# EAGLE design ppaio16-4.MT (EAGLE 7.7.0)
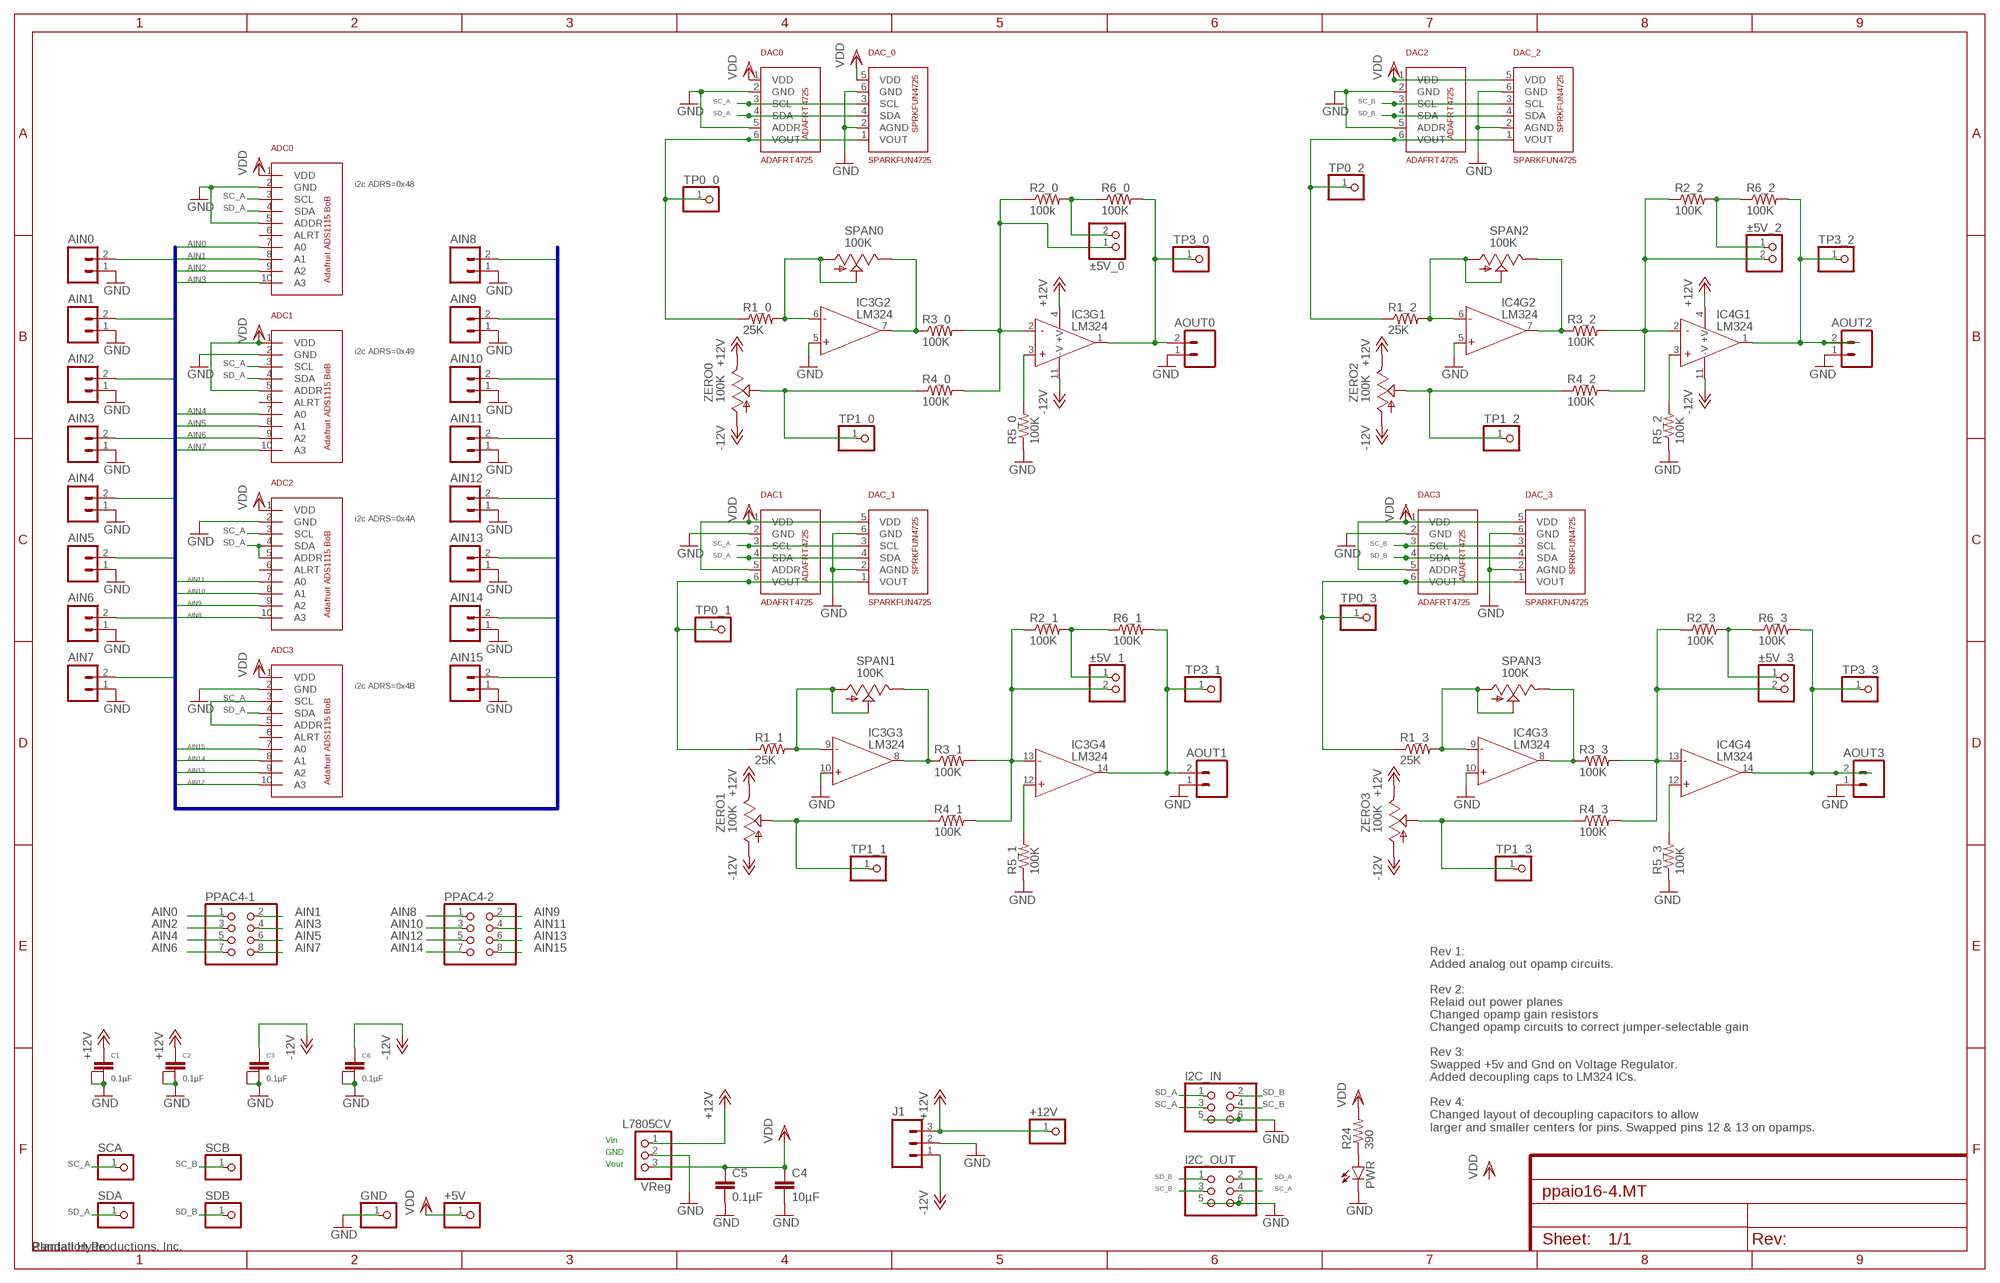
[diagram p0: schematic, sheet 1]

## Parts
+5V  PINHD-1X1  [1X01]
+12V  PINHD-1X1  [1X01]
ADC0  ADAFRTADS1115  [SIL10]
ADC1  ADAFRTADS1115  [SIL10]
ADC2  ADAFRTADS1115  [SIL10]
ADC3  ADAFRTADS1115  [SIL10]
AIN0  M025MM  [SCREWTERMINAL-5MM-2]
AIN1  M025MM  [SCREWTERMINAL-5MM-2]
AIN2  M025MM  [SCREWTERMINAL-5MM-2]
AIN3  M025MM  [SCREWTERMINAL-5MM-2]
AIN4  M025MM  [SCREWTERMINAL-5MM-2]
AIN5  M025MM  [SCREWTERMINAL-5MM-2]
AIN6  M025MM  [SCREWTERMINAL-5MM-2]
AIN7  M025MM  [SCREWTERMINAL-5MM-2]
AIN8  M025MM  [SCREWTERMINAL-5MM-2]
AIN9  M025MM  [SCREWTERMINAL-5MM-2]
AIN10  M025MM  [SCREWTERMINAL-5MM-2]
AIN11  M025MM  [SCREWTERMINAL-5MM-2]
AIN12  M025MM  [SCREWTERMINAL-5MM-2]
AIN13  M025MM  [SCREWTERMINAL-5MM-2]
AIN14  M025MM  [SCREWTERMINAL-5MM-2]
AIN15  M025MM  [SCREWTERMINAL-5MM-2]
AOUT0  M025MM  [SCREWTERMINAL-5MM-2]
AOUT1  M025MM  [SCREWTERMINAL-5MM-2]
AOUT2  M025MM  [SCREWTERMINAL-5MM-2]
AOUT3  M025MM  [SCREWTERMINAL-5MM-2]
C1  0.1µF  CAPACITOR  [1+2CAP]
C2  0.1µF  CAPACITOR  [1+2CAP]
C3  0.1µF  CAPACITOR  [1+2CAP]
C4  10µF  C2.5/2  [C2.5-2]
C5  0.1µF  C2.5/2  [C2.5-2]
C6  0.1µF  CAPACITOR  [1+2CAP]
DAC0  ADAFRT4725  [SIL6]
DAC1  ADAFRT4725  [SIL6]
DAC2  ADAFRT4725  [SIL6]
DAC3  ADAFRT4725  [SIL6]
DAC_0  SPARKFUN4725  [SIL6]
DAC_1  SPARKFUN4725  [SIL6]
DAC_2  SPARKFUN4725  [SIL6]
DAC_3  SPARKFUN4725  [SIL6]
FRAME1  FRAME_11X17_CU_MARK  [FR-LTR-ON-PCB]
GND  PINHD-1X1  [1X01]
I2C_IN  PINHD-2X3  [2X03]
I2C_OUT  PINHD-2X3  [2X03]
IC3  LM324  [DIL14]
IC4  LM324  [DIL14]
J1  M03-SCREW-5MM  [SCREWTERMINAL-5MM-3]
L7805CV  VReg  PINHD-1X3  [1X03]
PPAC4-1  PINHD-2X4  [2X04]
PPAC4-2  PINHD-2X4  [2X04]
PWR  LED5MM  [LED5MM]
R1_0  25K  10OHM-1/4W-5%(PTH)  [AXIAL-0.3]
R1_1  25K  10OHM-1/4W-5%(PTH)  [AXIAL-0.3]
R1_2  25K  10OHM-1/4W-5%(PTH)  [AXIAL-0.3]
R1_3  25K  10OHM-1/4W-5%(PTH)  [AXIAL-0.3]
R2_0  100k  10OHM-1/4W-5%(PTH)  [AXIAL-0.3]
R2_1  100K  10OHM-1/4W-5%(PTH)  [AXIAL-0.3]
R2_2  100K  10OHM-1/4W-5%(PTH)  [AXIAL-0.3]
R2_3  100K  10OHM-1/4W-5%(PTH)  [AXIAL-0.3]
R3_0  100K  10OHM-1/4W-5%(PTH)  [AXIAL-0.3]
R3_1  100K  10OHM-1/4W-5%(PTH)  [AXIAL-0.3]
R3_2  100K  10OHM-1/4W-5%(PTH)  [AXIAL-0.3]
R3_3  100K  10OHM-1/4W-5%(PTH)  [AXIAL-0.3]
R4_0  100K  10OHM-1/4W-5%(PTH)  [AXIAL-0.3]
R4_1  100K  10OHM-1/4W-5%(PTH)  [AXIAL-0.3]
R4_2  100K  10OHM-1/4W-5%(PTH)  [AXIAL-0.3]
R4_3  100K  10OHM-1/4W-5%(PTH)  [AXIAL-0.3]
R5_0  100K  10OHM-1/4W-5%(PTH)  [AXIAL-0.3]
R5_1  100K  10OHM-1/4W-5%(PTH)  [AXIAL-0.3]
R5_2  100K  10OHM-1/4W-5%(PTH)  [AXIAL-0.3]
R5_3  100K  10OHM-1/4W-5%(PTH)  [AXIAL-0.3]
R6_0  100K  10OHM-1/4W-5%(PTH)  [AXIAL-0.3]
R6_1  100K  10OHM-1/4W-5%(PTH)  [AXIAL-0.3]
R6_2  100K  10OHM-1/4W-5%(PTH)  [AXIAL-0.3]
R6_3  100K  10OHM-1/4W-5%(PTH)  [AXIAL-0.3]
R24  390  1KOHM-1/4W-1%(PTH)  [AXIAL-0.3]
SCA  PINHD-1X1  [1X01]
SCB  PINHD-1X1  [1X01]
SDA  PINHD-1X1  [1X01]
SDB  PINHD-1X1  [1X01]
SPAN0  100K  TRIM_US-B64Y  [B64Y]
SPAN1  100K  TRIM_US-B64Y  [B64Y]
SPAN2  100K  TRIM_US-B64Y  [B64Y]
SPAN3  100K  TRIM_US-B64Y  [B64Y]
TP0_0  PINHD-1X1  [1X01]
TP0_1  PINHD-1X1  [1X01]
TP0_2  PINHD-1X1  [1X01]
TP0_3  PINHD-1X1  [1X01]
TP1_0  PINHD-1X1  [1X01]
TP1_1  PINHD-1X1  [1X01]
TP1_2  PINHD-1X1  [1X01]
TP1_3  PINHD-1X1  [1X01]
TP3_0  PINHD-1X1  [1X01]
TP3_1  PINHD-1X1  [1X01]
TP3_2  PINHD-1X1  [1X01]
TP3_3  PINHD-1X1  [1X01]
ZERO0  100K  TRIM_US-B64Y  [B64Y]
ZERO1  100K  TRIM_US-B64Y  [B64Y]
ZERO2  100K  TRIM_US-B64Y  [B64Y]
ZERO3  100K  TRIM_US-B64Y  [B64Y]
±5V_0  PINHD-1X2  [1X02]
±5V_1  PINHD-1X2  [1X02]
±5V_2  PINHD-1X2  [1X02]
±5V_3  PINHD-1X2  [1X02]

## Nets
+12V [RelayConn]: +12V.1 C1.1 C2.1 IC3.4(+V) IC4.4(+V) J1.3 L7805CV.1 ZERO0.E ZERO1.E ZERO2.E ZERO3.E
-12V [RelayConn]: C3.1 C6.1 IC3.11(-V) IC4.11(-V) J1.1 ZERO0.A ZERO1.A ZERO2.A ZERO3.A
AIN0: ADC0.7(A0) AIN0.2 PPAC4-1.1
AIN1: ADC0.8(A1) AIN1.2 PPAC4-1.2
AIN2: ADC0.9(A2) AIN2.2 PPAC4-1.3
AIN3: ADC0.10(A3) AIN3.2 PPAC4-1.4
AIN4: ADC1.7(A0) AIN4.2 PPAC4-1.5
AIN5: ADC1.8(A1) AIN5.2 PPAC4-1.6
AIN6: ADC1.9(A2) AIN6.2 PPAC4-1.7
AIN7: ADC1.10(A3) AIN7.2 PPAC4-1.8
AIN8: ADC2.10(A3) AIN8.2 PPAC4-2.1
AIN9: ADC2.9(A2) AIN9.2 PPAC4-2.2
AIN10: ADC2.8(A1) AIN10.2 PPAC4-2.3
AIN11: ADC2.7(A0) AIN11.2 PPAC4-2.4
AIN12: ADC3.10(A3) AIN12.2 PPAC4-2.5
AIN13: ADC3.9(A2) AIN13.2 PPAC4-2.6
AIN14: ADC3.8(A1) AIN14.2 PPAC4-2.7
AIN15: ADC3.7(A0) AIN15.2 PPAC4-2.8
GND [Ground]: ADC0.2(GND) ADC0.5(ADDR) ADC1.2(GND) ADC2.2(GND) ADC3.2(GND) AIN0.1 AIN1.1 AIN2.1 AIN3.1 AIN4.1 AIN5.1 AIN6.1 AIN7.1 AIN8.1 AIN9.1 AIN10.1 AIN11.1 AIN12.1 AIN13.1 AIN14.1 AIN15.1 AOUT0.1 AOUT1.1 AOUT2.1 AOUT3.1 C1.2@1 C1.2@2 C2.2@1 C2.2@2 C3.2@1 C3.2@2 C4.2 C5.2 C6.2@1 C6.2@2 DAC0.2(GND) DAC0.5(ADDR) DAC1.2(GND) DAC2.2(GND) DAC2.5(ADDR) DAC3.2(GND) DAC_0.2(AGND) DAC_0.6(GND) DAC_1.2(AGND) DAC_1.6(GND) DAC_2.2(AGND) DAC_2.6(GND) DAC_3.2(AGND) DAC_3.6(GND) GND.1 I2C_IN.5 I2C_IN.6 I2C_OUT.5 I2C_OUT.6 IC3.5(+IN) IC3.10(+IN) IC4.5(+IN) IC4.10(+IN) J1.2 L7805CV.2 PWR.K(C) R5_0.P$1 R5_1.P$1 R5_2.P$1 R5_3.P$1
N$1: DAC0.6(VOUT) DAC_0.1(VOUT) R1_0.P$1 TP0_0.1
N$2: DAC1.6(VOUT) DAC_1.1(VOUT) R1_1.P$1 TP0_1.1
N$3: DAC2.6(VOUT) DAC_2.1(VOUT) R1_2.P$1 TP0_2.1
N$4: DAC3.6(VOUT) DAC_3.1(VOUT) R1_3.P$1 TP0_3.1
N$5: AOUT0.2 IC3.1(OUT) R6_0.P$2 TP3_0.1
N$6: R2_1.P$2 R6_1.P$1 ±5V_1.1
N$7: R2_3.P$2 R6_3.P$1 ±5V_3.1
N$8: R2_2.P$2 R6_2.P$1 ±5V_2.1
N$9: R2_0.P$2 R6_0.P$1 ±5V_0.2
N$10: IC3.12(+IN) R5_1.P$2
N$11: IC4.12(+IN) R5_3.P$2
N$26: PWR.A R24.P$1
N$38: IC3.6(-IN) R1_0.P$2 SPAN0.A SPAN0.S
N$39: IC3.7(OUT) R3_0.P$1 SPAN0.E
N$40: IC3.2(-IN) R2_0.P$1 R3_0.P$2 R4_0.P$2 ±5V_0.1
N$42: R4_0.P$1 TP1_0.1 ZERO0.S
N$45: IC3.9(-IN) R1_1.P$2 SPAN1.A SPAN1.S
N$46: IC3.8(OUT) R3_1.P$1 SPAN1.E
N$47: IC3.13(-IN) R2_1.P$1 R3_1.P$2 R4_1.P$2 ±5V_1.2
N$48: AOUT1.2 IC3.14(OUT) R6_1.P$2 TP3_1.1
N$49: R4_1.P$1 TP1_1.1 ZERO1.S
N$52: IC3.3(+IN) R5_0.P$2
N$54: IC4.6(-IN) R1_2.P$2 SPAN2.A SPAN2.S
N$55: IC4.7(OUT) R3_2.P$1 SPAN2.E
N$56: IC4.2(-IN) R2_2.P$1 R3_2.P$2 R4_2.P$2 ±5V_2.2
N$57: AOUT2.2 IC4.1(OUT) R6_2.P$2 TP3_2.1
N$58: R4_2.P$1 TP1_2.1 ZERO2.S
N$61: IC4.9(-IN) R1_3.P$2 SPAN3.A SPAN3.S
N$62: IC4.8(OUT) R3_3.P$1 SPAN3.E
N$63: IC4.13(-IN) R2_3.P$1 R3_3.P$2 R4_3.P$2 ±5V_3.2
N$64: AOUT3.2 IC4.14(OUT) R6_3.P$2 TP3_3.1
N$65: R4_3.P$1 TP1_3.1 ZERO3.S
N$68: IC4.3(+IN) R5_2.P$2
SC_A: ADC0.3(SCL) ADC1.3(SCL) ADC2.3(SCL) ADC3.3(SCL) ADC3.5(ADDR) DAC0.3(SCL) DAC1.3(SCL) DAC_0.3(SCL) DAC_1.3(SCL) I2C_IN.3 I2C_OUT.4 SCA.1
SC_B: DAC2.3(SCL) DAC3.3(SCL) DAC_2.3(SCL) DAC_3.3(SCL) I2C_IN.4 I2C_OUT.3 SCB.1
SD_A: ADC0.4(SDA) ADC1.4(SDA) ADC2.4(SDA) ADC2.5(ADDR) ADC3.4(SDA) DAC0.4(SDA) DAC1.4(SDA) DAC_0.4(SDA) DAC_1.4(SDA) I2C_IN.1 I2C_OUT.2 SDA.1
SD_B: DAC2.4(SDA) DAC3.4(SDA) DAC_2.4(SDA) DAC_3.4(SDA) I2C_IN.2 I2C_OUT.1 SDB.1
VDD: +5V.1 ADC0.1(VDD) ADC1.1(VDD) ADC1.5(ADDR) ADC2.1(VDD) ADC3.1(VDD) C4.1 C5.1 DAC0.1(VDD) DAC1.1(VDD) DAC1.5(ADDR) DAC2.1(VDD) DAC3.1(VDD) DAC3.5(ADDR) DAC_0.5(VDD) DAC_1.5(VDD) DAC_2.5(VDD) DAC_3.5(VDD) L7805CV.3 R24.P$2
Unconnected: ADC0.6(ALRT) ADC1.6(ALRT) ADC2.6(ALRT) ADC3.6(ALRT)

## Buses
ABUS:AIN[0..15]

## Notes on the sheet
- i2c ADRS=0x48
- i2c ADRS=0x49
- i2c ADRS=0x4A
- i2c ADRS=0x4B
- Rev 1:
  Added analog out opamp circuits.
  
  Rev 2:
  Relaid out power planes
  Changed opamp gain resistors
  Changed opamp circuits to correct jumper-selectable gain
  
  Rev 3:
  Swapped +5v and Gnd on Voltage Regulator.
  Added decoupling caps to LM324 ICs.
  
  Rev 4:
  Changed layout of decoupling capacitors to allow
  larger and smaller centers for pins. Swapped pins 12 & 13 on opamps.
- Vin
- GND
- Vout

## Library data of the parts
+5V +12V GND SCA SCB SDA SDB TP0_0 TP0_1-TP0_3 TP1_0 TP1_1-TP1_3 TP3_0 TP3_1-TP3_3 = pinhead:PINHD-1X1: PIN HEADER
ADC0 ADC1-ADC3 = PlantProd:ADAFRTADS1115: Adafruit ADS1115 16-bit ADC breakout board
AIN0 AIN1-AIN15 AOUT0 AOUT1-AOUT3 = SparkFun-Connectors:M02: Standard 2-pin 0.1" header. Use with; STOREFRONT_ID: PRT-08432
C1-C3 C6 = PlantProd:CAPACITOR: Capacitor with three terminals to support multiple capacitor sizes.
C4 C5 = capacitor-wima:C: CAPACITOR
DAC0 DAC1-DAC3 = PlantProd:ADAFRT4725: ADAFRT4725 - MCP4725 12-bit DAC BoB
DAC_0 DAC_1-DAC_3 = PlantProd:SPARKFUN4725: ADAFRT4725 - MCP4725 12-bit DAC BoB
FRAME1 = ProperFrame:FRAME_11X17_CU_MARK: Frame sized for 11x17" page with 0.25" margin. Places name, datecode and revision mark in bottom copper layer of PCB.; CNAME: Plantation Productions, Inc.; CREVISION: 2; DESIGNER: Randall Hyde
I2C_IN I2C_OUT = pinhead:PINHD-2X3: PIN HEADER
IC3 IC4 = PlantProd:LM324: LM324 quad op-amp
J1 = SparkFun-Connectors:M03: Header 3 Standard 3-pin 0.1" header. Use with straight break away headers (SKU : PRT-00116), right angle break away headers (PRT-00553), swiss pins (PRT-00743), machine pins (PRT-00117), and female headers (PRT-00115). Molex polarized connector foot print use with SKU : PRT-08232 with associated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; STOREFRONT_ID: PRT-08433
L7805CV = pinhead:PINHD-1X3: PIN HEADER
PPAC4-1 PPAC4-2 = pinhead:PINHD-2X4: PIN HEADER
PWR = SparkFun-LED:LED: LEDs
R1_0 R1_1-R1_3 R2_0 R2_1-R2_3 R3_0 R3_1-R3_3 R4_0 R4_1-R4_3 R5_0 R5_1-R5_3 R6_0 R6_1-R6_3 = SparkFun-Resistors:10OHM-1/4W-5%(PTH): RES-10698; PROD_ID: RES-10698; VALUE: 10
R24 = SparkFun-Resistors:1KOHM-1/4W-1%(PTH): RES-12182; PROD_ID: RES-12182; VALUE: 1K
SPAN0 SPAN1-SPAN3 ZERO0 ZERO1-ZERO3 = pot:TRIM_US-: POTENTIOMETER
±5V_0 ±5V_1-±5V_3 = pinhead:PINHD-1X2: PIN HEADER

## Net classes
1 Ground: width 0.762 mm, drill 1 mm, clearance 0.102 mm
2 RelayConn: width 0.762 mm, drill 0.025 mm, clearance 0.508 mm
3 HiCurSignal: width 0.762 mm, drill 0.025 mm, clearance 0.102 mm

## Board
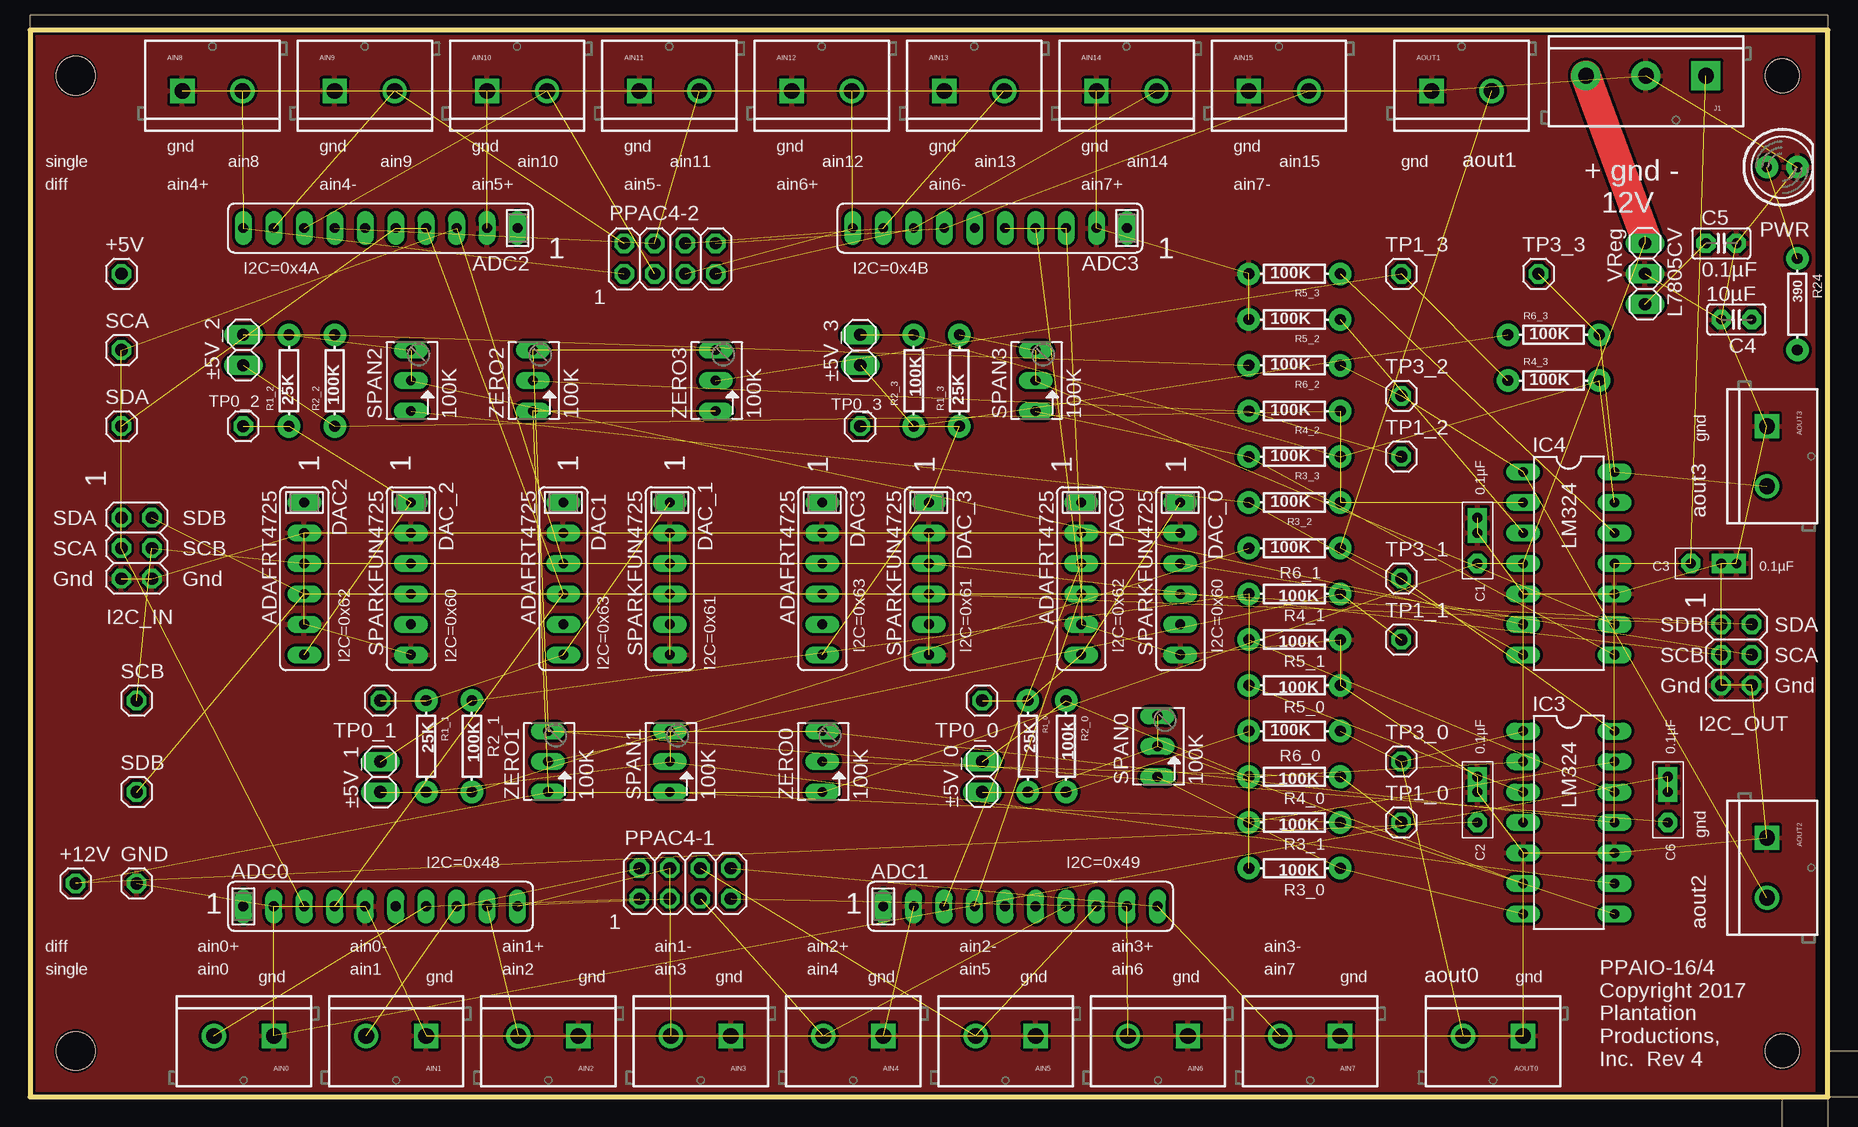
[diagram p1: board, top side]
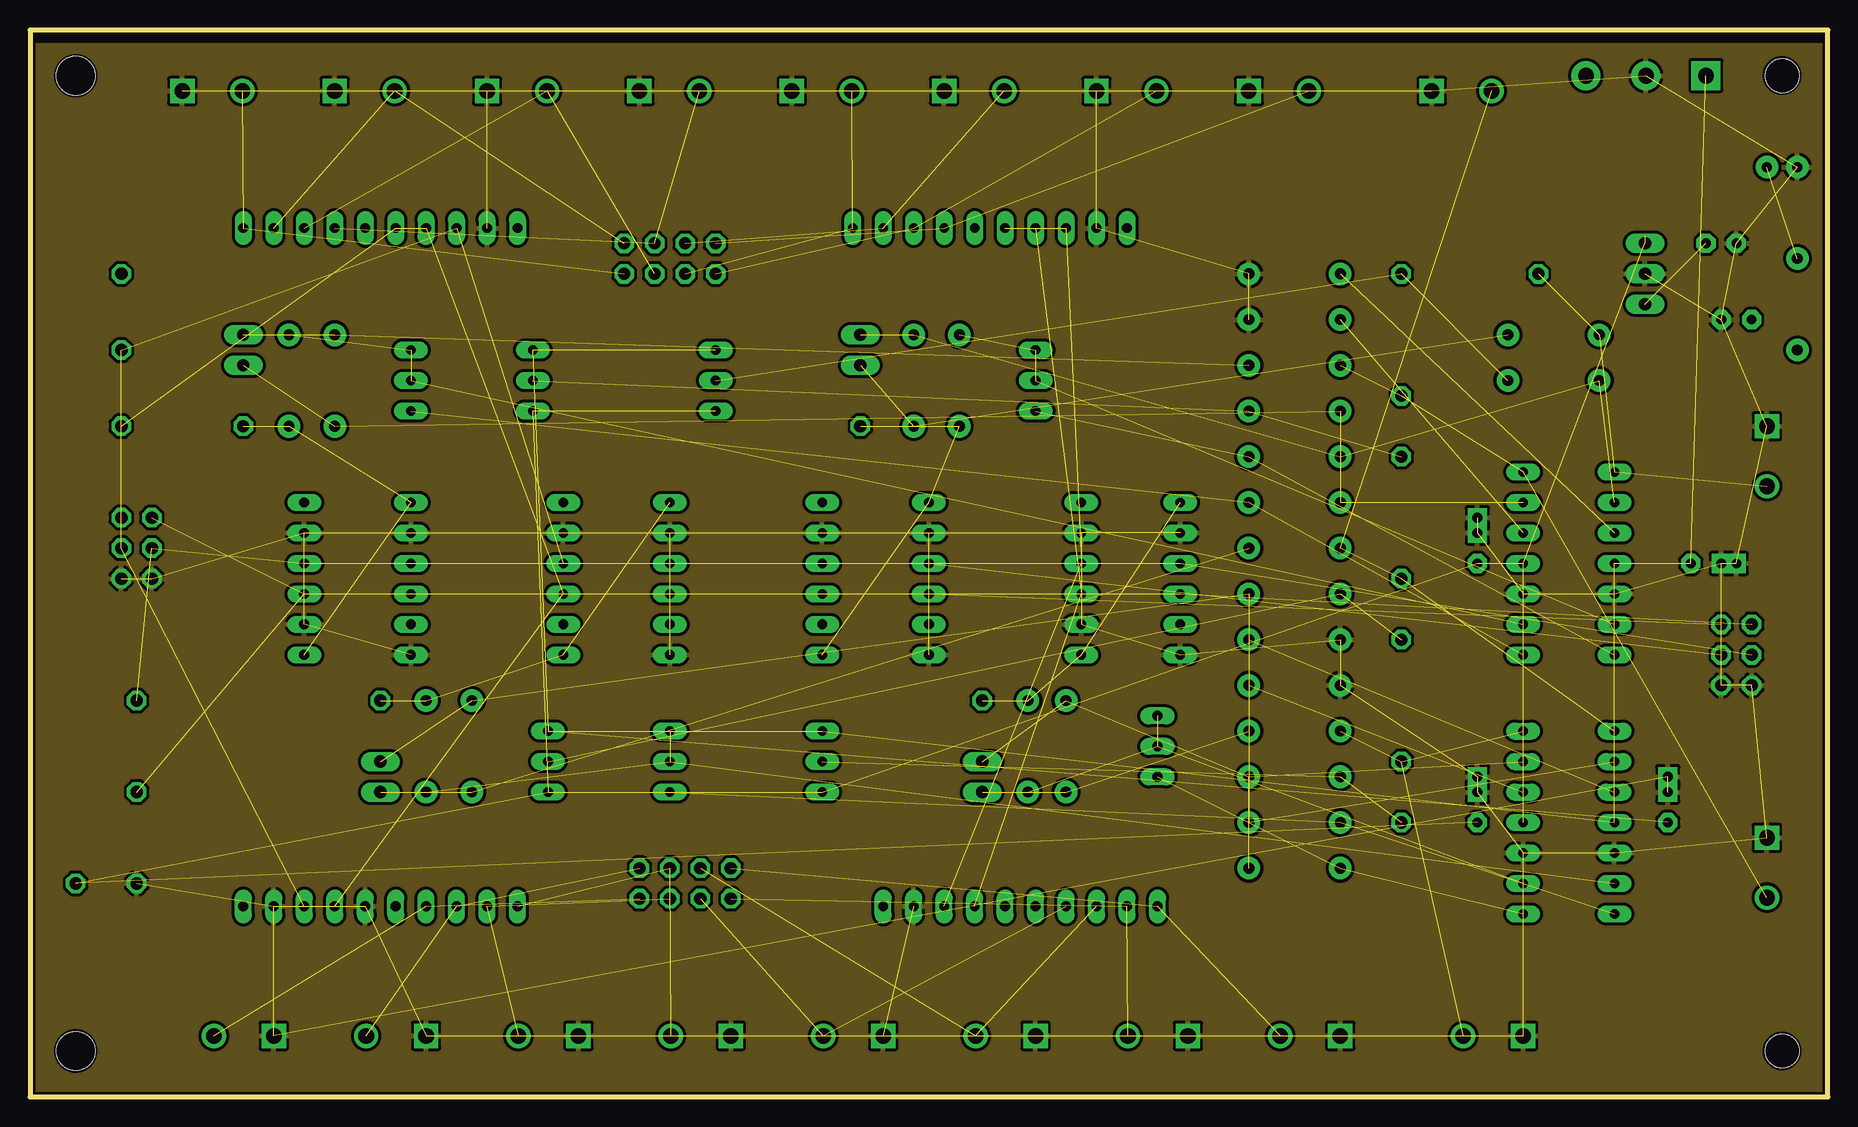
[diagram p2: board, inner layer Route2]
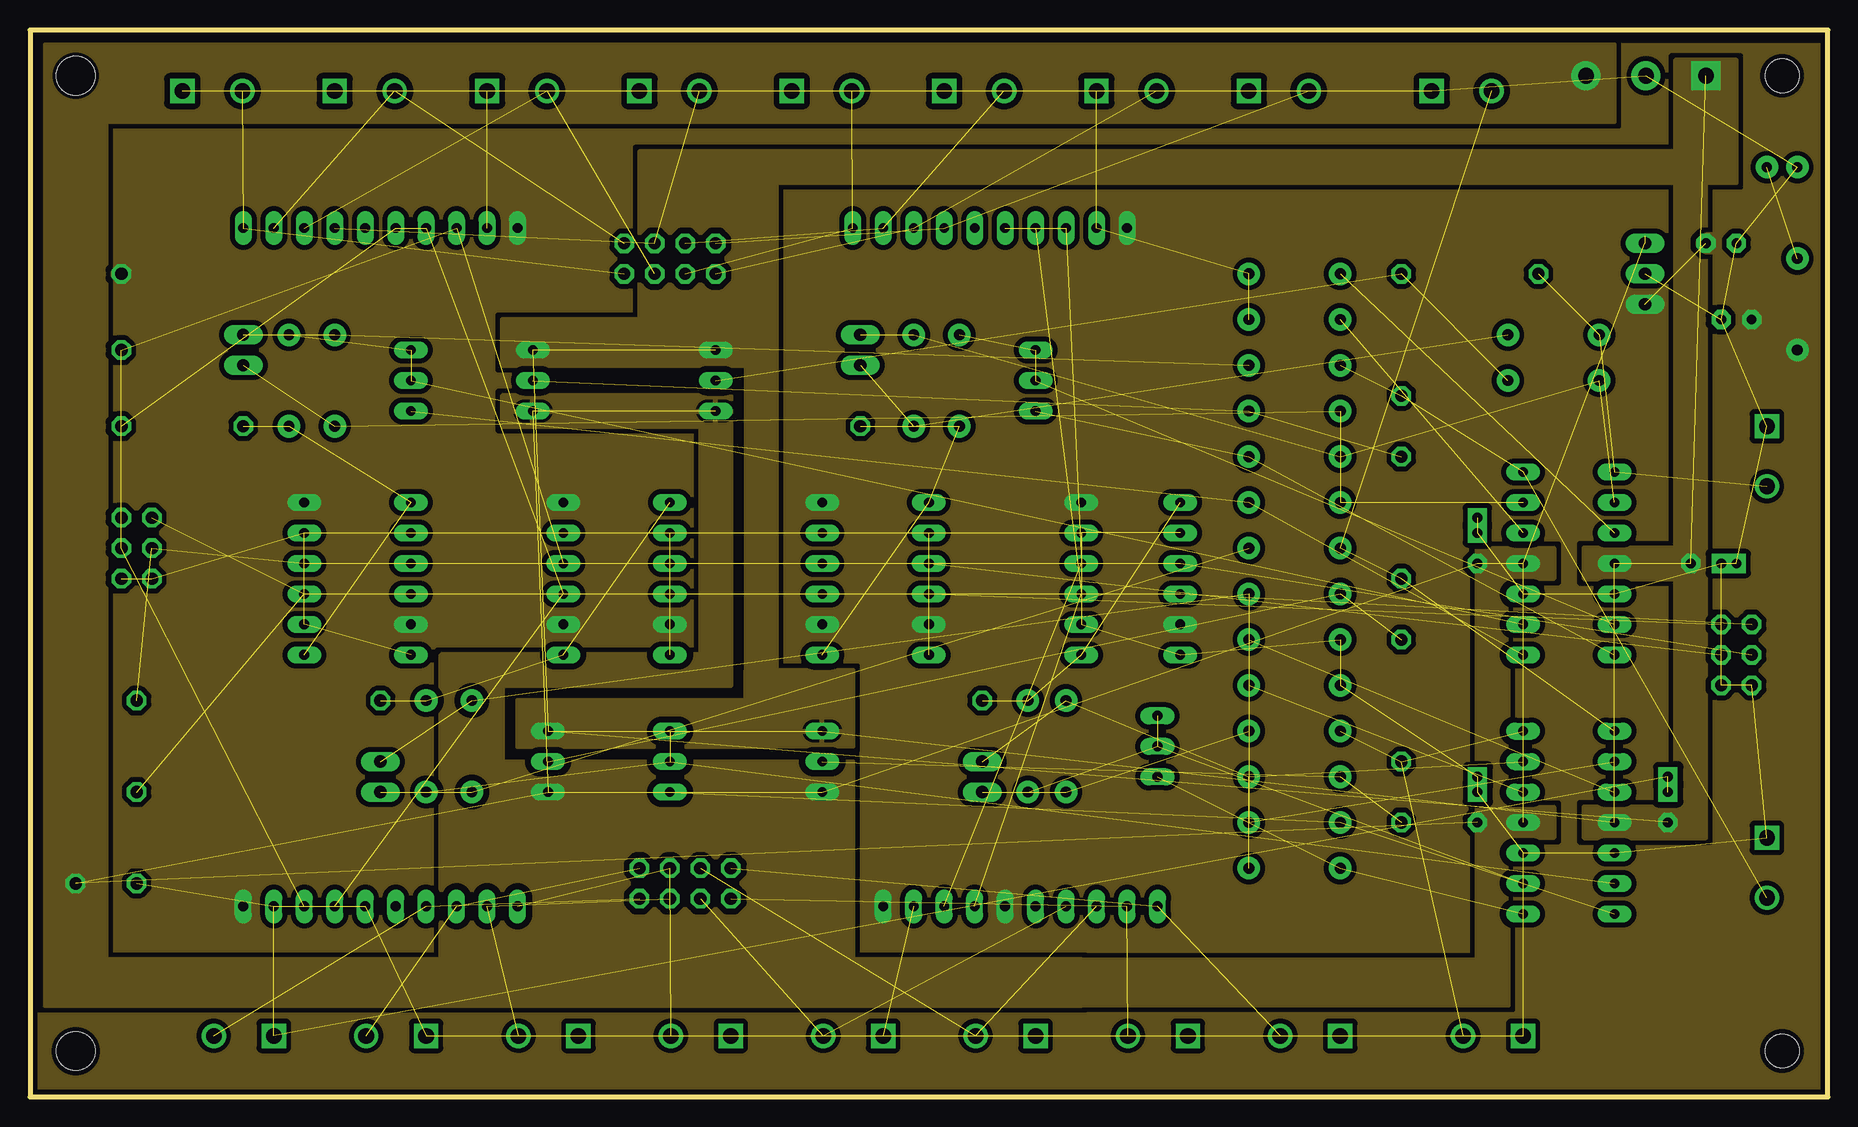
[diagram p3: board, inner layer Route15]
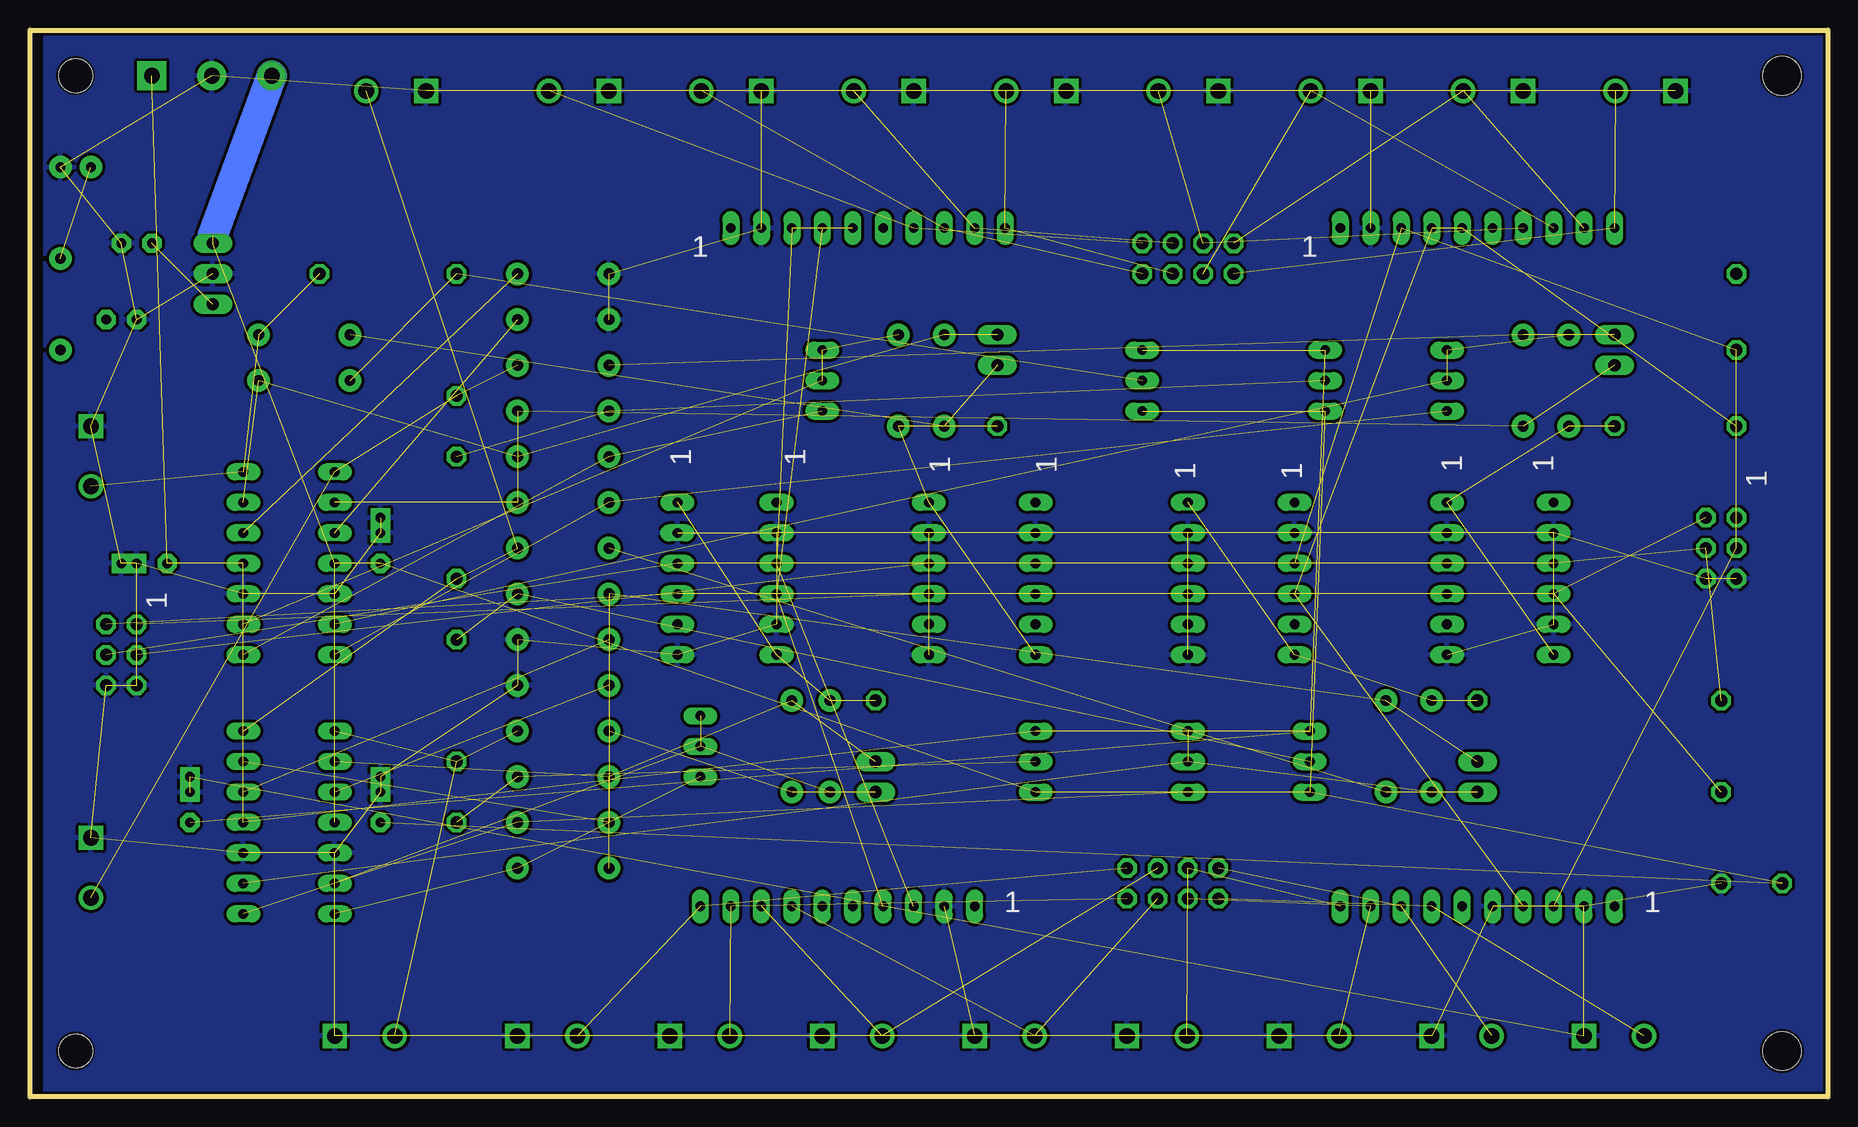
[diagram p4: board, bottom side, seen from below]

Size 149.86 x 88.9 mm. Coordinates in mm from the lower left corner, seen from the top.
Outline: 0,0 149.86,0 149.86,88.9 0,88.9 0,0
Copper layers (1*2*15*16): Top 0.035mm / dielectric 1.5mm / Route2 0.035mm / dielectric 0.15mm / Route15 0.035mm / dielectric 0.2mm / Bottom 0.035mm
Design rules "SeeedStudio_2layer_DRU_no_angle_20140221 *": minimum track width 10mil, minimum drill 20mil, track to track 10mil, track to pad 10mil, pad to pad 10mil, via to via 10mil, smd to smd 8mil, copper to edge 8mil, drill to drill 8mil, minimum pad ring 12mil, minimum via ring 10mil, stop-mask expansion 4mil, vias tented up to drill 25mil, thermal gap 10mil
Holes 3.2 mm at 3.81,85.09 3.81,3.81
Holes 2.8 mm at 146.05,85.09 146.05,3.81

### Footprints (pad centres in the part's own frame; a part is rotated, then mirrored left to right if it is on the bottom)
1X01 = drill 1.016 octagon: 1 0,0
SIL10 = drill 0.813 long: 1 -10.16,0; 2 -7.62,0; 3 -5.08,0; 4 -2.54,0; 5 0,0; 6 2.54,0; 7 5.08,0; 8 7.62,0; 9 10.16,0; 10 12.7,0
SCREWTERMINAL-5MM-2 = drill 1.3 pad 2.032 square: 1 0,0 | drill 1.3 pad 2.032: 2 5,0
1+2CAP = drill 0.813 pad 1.6 octagon: 1 -2.54,0 | drill 0.813 pad 1.6 square: 2@1 0,0; 2@2 1.27,0
C2.5-2 = drill 0.813 pad 1.6 octagon: 1 -1.27,0; 2 1.27,0
SIL6 = drill 0.813 long: 1 -10.16,0; 2 -7.62,0; 3 -5.08,0; 4 -2.54,0; 5 0,0; 6 2.54,0
2X03 = drill 1.016 octagon: 1 -2.54,-1.27; 2 -2.54,1.27; 3 0,-1.27; 4 0,1.27; 5 2.54,-1.27; 6 2.54,1.27
DIL14 = drill 0.813 long: 1 -7.62,-3.81; 2 -5.08,-3.81; 3 -2.54,-3.81; 4 0,-3.81; 5 2.54,-3.81; 6 5.08,-3.81; 7 7.62,-3.81; 8 7.62,3.81; 9 5.08,3.81; 10 2.54,3.81; 11 0,3.81; 12 -2.54,3.81; 13 -5.08,3.81; 14 -7.62,3.81
SCREWTERMINAL-5MM-3 = drill 1.3 pad 2.413 square: 1 0,0 | drill 1.3 pad 2.413: 2 5,0; 3 10,0
1X03 = drill 1.016 long: 1 -2.54,0; 2 0,0; 3 2.54,0
2X04 = drill 1.016 octagon: 1 -3.81,-1.27; 2 -3.81,1.27; 3 -1.27,-1.27; 4 -1.27,1.27; 5 1.27,-1.27; 6 1.27,1.27; 7 3.81,-1.27; 8 3.81,1.27
LED5MM = drill 0.813 pad 1.88: A -1.27,0; K 1.27,0
AXIAL-0.3 = drill 0.9 pad 1.88: P$1 -3.81,0; P$2 3.81,0
B64Y = drill 0.813 long: A 2.54,0; E -2.54,0; S 0,0
1X02 = drill 1.016 long: 1 -1.27,0; 2 1.27,0

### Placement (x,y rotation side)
+5V  7.62,68.58 0 top
+12V  3.81,17.78 0 top
ADC0  27.94,15.88 0 top
ADC1  81.28,15.88 0 top
ADC2  30.48,72.39 180 top
ADC3  81.28,72.39 180 top
AIN0  20.32,5.08 180 top
AIN1  33.02,5.08 180 top
AIN2  45.72,5.08 180 top
AIN3  58.42,5.08 180 top
AIN4  71.12,5.08 180 top
AIN5  83.82,5.08 180 top
AIN6  96.52,5.08 180 top
AIN7  109.22,5.08 180 top
AIN8  12.7,83.82 0 top
AIN9  25.4,83.82 0 top
AIN10  38.1,83.82 0 top
AIN11  50.8,83.82 0 top
AIN12  63.5,83.82 0 top
AIN13  76.2,83.82 0 top
AIN14  88.9,83.82 0 top
AIN15  101.6,83.82 0 top
AOUT0  124.46,5.08 180 top
AOUT1  116.84,83.82 0 top
AOUT2  144.78,21.59 270 top
AOUT3  144.78,55.88 270 top
C1  120.65,46.99 90 top
C2  120.65,25.4 90 top
C3  140.97,44.45 0 top
C4  142.24,64.77 180 top
C5  140.97,71.12 0 top
C6  136.53,25.4 90 top
DAC0  87.63,39.37 270 top
DAC1  44.45,39.37 270 top
DAC2  22.86,39.37 270 top
DAC3  66.04,39.37 270 top
DAC_0  95.89,39.37 270 top
DAC_1  53.34,39.37 270 top
DAC_2  31.75,39.37 270 top
DAC_3  74.93,39.37 270 top
FRAME1  not placed on the board
GND  8.89,17.78 0 top
I2C_IN  8.89,45.72 270 top
I2C_OUT  142.24,36.83 270 top
IC3  128.27,22.86 270 top
IC4  128.27,44.45 270 top
J1  139.7,85.09 180 top
L7805CV  134.62,68.58 270 top
PPAC4-1  54.61,17.78 0 top
PPAC4-2  53.34,69.85 0 top
PWR  146.05,77.47 0 top
R1_0  83.19,29.21 270 top
R1_1  33.02,29.21 270 top
R1_2  21.59,59.69 90 top
R1_3  77.47,59.69 90 top
R2_0  86.36,29.21 270 top
R2_1  36.83,29.21 270 top
R2_2  25.4,59.69 90 top
R2_3  73.66,59.69 270 top
R3_0  105.41,19.05 180 top
R3_1  105.41,22.86 180 top
R3_2  105.41,49.53 0 top
R3_3  105.41,53.34 0 top
R4_0  105.41,26.67 180 top
R4_1  105.41,41.91 180 top
R4_2  105.41,57.15 0 top
R4_3  127,59.69 0 top
R5_0  105.41,34.29 180 top
R5_1  105.41,38.1 180 top
R5_2  105.41,64.77 0 top
R5_3  105.41,68.58 0 top
R6_0  105.41,30.48 0 top
R6_1  105.41,45.72 0 top
R6_2  105.41,60.96 0 top
R6_3  127,63.5 0 top
R24  147.32,66.04 270 top
SCA  7.62,62.23 0 top
SCB  8.89,33.02 0 top
SDA  7.62,55.88 0 top
SDB  8.89,25.4 0 top
SPAN0  93.98,29.21 90 top
SPAN1  53.34,27.94 90 top
SPAN2  31.75,59.69 90 top
SPAN3  83.82,59.69 90 top
TP0_0  79.38,33.02 180 top
TP0_1  29.21,33.02 180 top
TP0_2  17.78,55.88 180 top
TP0_3  69.22,55.88 180 top
TP1_0  114.3,22.86 0 top
TP1_1  114.3,38.1 0 top
TP1_2  114.3,53.34 0 top
TP1_3  114.3,68.58 0 top
TP3_0  114.3,27.94 0 top
TP3_1  114.3,43.18 0 top
TP3_2  114.3,58.42 0 top
TP3_3  125.73,68.58 0 top
ZERO0  66.04,27.94 90 top
ZERO1  43.18,27.94 90 top
ZERO2  41.91,59.69 90 top
ZERO3  57.15,59.69 90 top
±5V_0  79.38,26.67 270 top
±5V_1  29.21,26.67 90 top
±5V_2  17.78,62.23 270 top
±5V_3  69.22,62.23 90 top

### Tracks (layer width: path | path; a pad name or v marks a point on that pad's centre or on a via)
+12V  (10 unrouted)
  Top 2.54: J1.3 134.62,71.75
  Bottom 2.54: J1.3 134.62,71.75
  pour Route15 (isolate 0.305, no thermals): 123.19,7.62 59.69,7.62 59.69,11.43 120.65,11.43 120.65,45.72 127,45.72 127,43.18 123.19,43.18 123.19,24.13 127,24.13 127,21.59 123.19,21.59
  pour Route15 (isolate 0.305, no thermals): 34.29,36.83 39.37,36.83 39.37,27.94 68.58,27.94 68.58,10.16 34.29,10.16
  pour Route15 (isolate 0.305, no thermals): 132.08,87.63 1.27,87.63 1.27,7.62 87.63,7.62 87.63,11.43 6.35,11.43 6.35,81.28 132.08,81.28
  pour Route15: 39.37,58.42 39.37,55.88 55.88,55.88 55.88,36.83 34.29,36.83 34.29,34.29 58.42,34.29 58.42,58.42
-12V  (8 unrouted)
  pour Route15 (isolate 0.305, no thermals): 137.16,86.36 137.16,78.74 50.8,78.74 50.8,64.77 39.37,64.77 39.37,60.96 59.69,60.96 59.69,33.02 40.64,33.02 40.64,29.21 62.23,29.21 62.23,76.2 142.24,76.2 142.24,86.36
  pour Route15 (isolate 0.305): 59.69,35.56 68.58,35.56 68.58,29.21 59.69,29.21
  pour Route15 (isolate 0.406, no thermals): 135.89,76.2 137.16,76.2 137.16,45.72 129.54,45.72 129.54,43.18 137.16,43.18 137.16,24.13 129.54,24.13 129.54,21.59 139.7,21.59 139.7,77.47 135.89,77.47
AIN0  (2 unrouted)
AIN1  (2 unrouted)
AIN2  (2 unrouted)
AIN3  (2 unrouted)
AIN4  (2 unrouted)
AIN5  (2 unrouted)
AIN6  (2 unrouted)
AIN7  (2 unrouted)
AIN8  (2 unrouted)
AIN9  (2 unrouted)
AIN10  (2 unrouted)
AIN11  (2 unrouted)
AIN12  (2 unrouted)
AIN13  (2 unrouted)
AIN14  (2 unrouted)
AIN15  (2 unrouted)
GND  (64 unrouted)
  pour Route2: 0,87.63 149.86,87.63 149.86,0 0,0
  pour Top: 0,88.9 148.59,88.9 148.59,0 0,0
  pour Bottom: 0,88.9 148.59,88.9 148.59,0 0,0
N$1  (3 unrouted)
N$2  (3 unrouted)
N$3  (3 unrouted)
N$4  (3 unrouted)
N$5  (3 unrouted)
N$6  (2 unrouted)
N$7  (2 unrouted)
N$8  (2 unrouted)
N$9  (2 unrouted)
N$10  (1 unrouted)
N$11  (1 unrouted)
N$26  (1 unrouted)
N$38  (3 unrouted)
N$39  (2 unrouted)
N$40  (4 unrouted)
N$42  (2 unrouted)
N$45  (3 unrouted)
N$46  (2 unrouted)
N$47  (4 unrouted)
N$48  (3 unrouted)
N$49  (2 unrouted)
N$52  (1 unrouted)
N$54  (3 unrouted)
N$55  (2 unrouted)
N$56  (4 unrouted)
N$57  (3 unrouted)
N$58  (2 unrouted)
N$61  (3 unrouted)
N$62  (2 unrouted)
N$63  (4 unrouted)
N$64  (3 unrouted)
N$65  (2 unrouted)
N$68  (1 unrouted)
SC_A  (11 unrouted)
SC_B  (6 unrouted)
SD_A  (11 unrouted)
SD_B  (6 unrouted)
VDD  (1 unrouted)
  pour Route15 (isolate 0.406, rank 3, no thermals): 0,87.63 149.86,87.63 149.86,0 0,0

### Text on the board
tPlace: gnd | gnd | gnd | gnd | gnd | gnd | gnd | gnd | single | ain8 | ain9 | ain10 | ain11 | ain12 | ain13 | ain14 | ain15 | gnd | aout1 | diff | ain4+ | ain4- | ain5+ | ain5- | ain6+ | ain6- | ain7+ | ain7- | + gnd - / 12V | 1 | 1 | I2C=0x4A | I2C=0x4B | 1 | gnd | 1 | 1 | 1 | 1 | 1 | 1 | 1 | 1 | 1 | SDA | SDB | aout3 | SCA | SCB | Gnd | Gnd | I2C=0x63 | I2C=0x61 | I2C=0x62 | I2C=0x60 | 1 | SDB | SDA | I2C=0x62 | I2C=0x60 | I2C=0x63 | I2C=0x61 | SCB | SCA | Gnd | Gnd | gnd | I2C=0x48 | I2C=0x49 | 1 | 1 | 1 | aout2 | diff | ain0+ | ain0- | ain1+ | ain1- | ain2+ | ain2- | ain3+ | ain3- | single | ain0 | gnd | ain1 | gnd | ain2 | gnd | ain3 | gnd | ain4 | gnd | ain5 | gnd | ain6 | gnd | ain7 | gnd | aout0 | gnd | PPAIO-16/4 / Copyright 2017 / Plantation / Productions, / Inc. Rev 4
bPlace: 1 | 1 | 1 | 1 | 1 | 1 | 1 | 1 | 1 | 1 | 1 | 1 | 1 | 1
